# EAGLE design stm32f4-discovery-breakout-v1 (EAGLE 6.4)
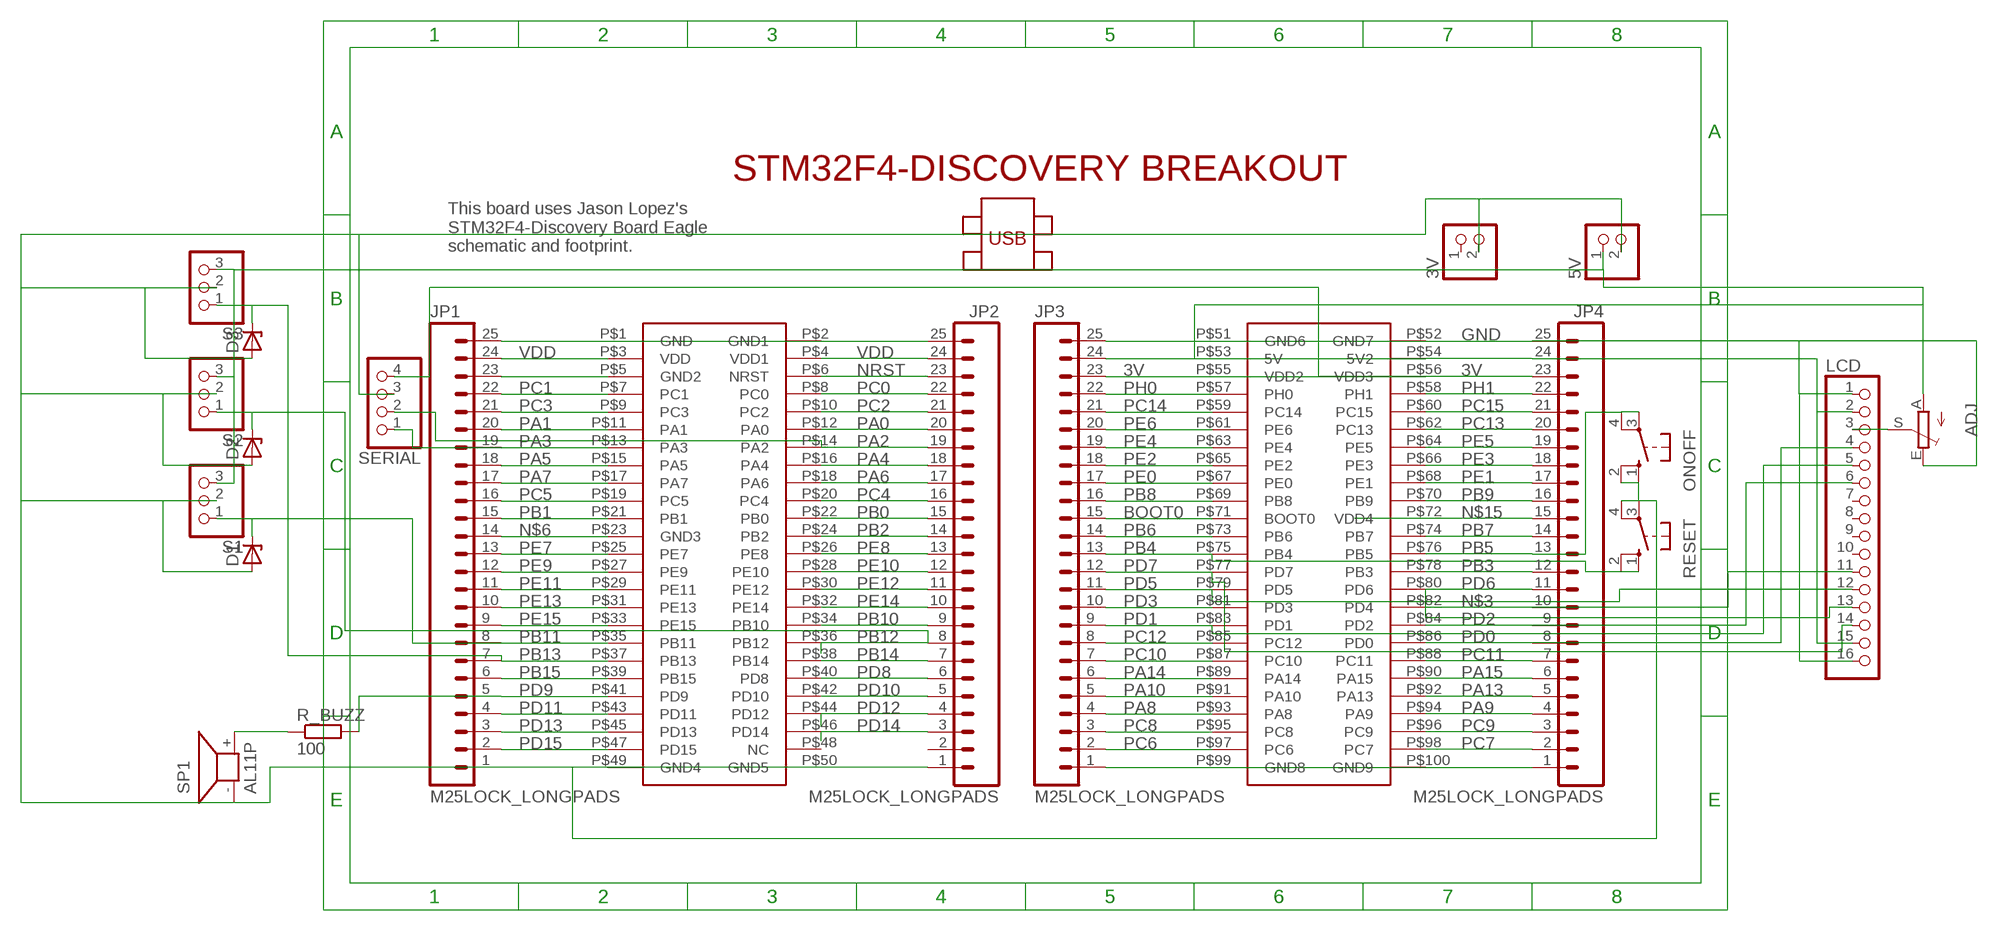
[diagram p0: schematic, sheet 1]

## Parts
3V  PINHD-1X2  [1X02]
5V  PINHD-1X2  [1X02]
ADJ  TRIM_EU-CA6V  [CA6V]
D1  ZENER-DIODEDO35Z10  [DO35Z10]
D2  ZENER-DIODEDO35Z10  [DO35Z10]
D3  ZENER-DIODEDO35Z10  [DO35Z10]
JP1  M25LOCK_LONGPADS  [1X25_LOCK_LONGPADS]
JP2  M25LOCK_LONGPADS  [1X25_LOCK_LONGPADS]
JP3  M25LOCK_LONGPADS  [1X25_LOCK_LONGPADS]
JP4  M25LOCK_LONGPADS  [1X25_LOCK_LONGPADS]
LCD  PINHD-1X16  [1X16]
ONOFF  10-XX  [B3F-10XX]
R_BUZZ  100  R-EU_0204/7  [0204/7]
RESET  10-XX  [B3F-10XX]
S1  PINHD-1X3  [1X03]
S2  PINHD-1X3  [1X03]
S3  PINHD-1X3  [1X03]
SERIAL  PINHD-1X4  [1X04]
SP1  AL11P  [AL11P]
U$1  STM32F4-DISCOVERY  [STM32F4-DISCOVERY]

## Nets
3V: JP3.23 JP4.23 SERIAL.4 U$1.P$55(VDD2) U$1.P$56(VDD3)
+5V: 3V.2 5V.2 D1.A D2.A D3.A JP1.1 JP2.1 ONOFF.1(S) ONOFF.2(S1) RESET.3(P) RESET.4(P1) S1.2 S2.2 S3.2 SERIAL.3 SP1.- U$1.P$49(GND4) U$1.P$50(GND5)
BOOT0: JP3.15 U$1.P$71(BOOT0)
GND: ADJ.E JP3.25 JP4.25 LCD.1 LCD.16 U$1.P$51(GND6) U$1.P$52(GND7)
N$1: R_BUZZ.1 SP1.+
N$2: ADJ.S LCD.3
N$3: JP4.10 LCD.11 U$1.P$82(PD4)
N$4: JP1.25 JP2.25 U$1.P$1(GND) U$1.P$2(GND1)
N$5: JP3.1 JP4.1 U$1.P$99(GND8) U$1.P$100(GND9)
N$6: JP1.14 U$1.P$23(GND3)
N$12: JP1.23 U$1.P$5(GND2)
N$13: 5V.1 ADJ.A JP3.24 JP4.24 LCD.2 LCD.15 S1.3 S2.3 S3.3 U$1.P$53(5V) U$1.P$54(5V2)
N$15: JP4.15 U$1.P$72(VDD4)
NRST: JP2.23 U$1.P$6(NRST)
PA0: JP2.20 U$1.P$12(PA0)
PA1: JP1.20 U$1.P$11(PA1)
PA2: JP2.19 SERIAL.2 U$1.P$14(PA2)
PA3: JP1.19 SERIAL.1 U$1.P$13(PA3)
PA4: JP2.18 U$1.P$16(PA4)
PA5: JP1.18 U$1.P$15(PA5)
PA6: JP2.17 U$1.P$18(PA6)
PA7: JP1.17 U$1.P$17(PA7)
PA8: JP3.4 U$1.P$93(PA8)
PA9: JP4.4 U$1.P$94(PA9)
PA10: JP3.5 U$1.P$91(PA10)
PA13: JP4.5 U$1.P$92(PA13)
PA14: JP3.6 U$1.P$89(PA14)
PA15: JP4.6 U$1.P$90(PA15)
PB0: JP2.15 U$1.P$22(PB0)
PB1: JP1.15 U$1.P$21(PB1)
PB2: JP2.14 U$1.P$24(PB2)
PB3: JP4.12 U$1.P$78(PB3)
PB4: JP3.13 RESET.1(S) RESET.2(S1) U$1.P$75(PB4)
PB5: JP4.13 ONOFF.3(P) ONOFF.4(P1) U$1.P$76(PB5)
PB6: JP3.14 U$1.P$73(PB6)
PB7: JP4.14 U$1.P$74(PB7)
PB8: JP3.16 U$1.P$69(PB8)
PB9: JP4.16 U$1.P$70(PB9)
PB10: JP2.9 U$1.P$34(PB10)
PB11: D1.C JP1.8 S1.1 U$1.P$35(PB11)
PB12: D2.C JP2.8 S2.1 U$1.P$36(PB12)
PB13: D3.C JP1.7 S3.1 U$1.P$37(PB13)
PB14: JP2.7 U$1.P$38(PB14)
PB15: JP1.6 U$1.P$39(PB15)
PC0: JP2.22 U$1.P$8(PC0)
PC1: JP1.22 U$1.P$7(PC1)
PC2: JP2.21 U$1.P$10(PC2)
PC3: JP1.21 U$1.P$9(PC3)
PC4: JP2.16 U$1.P$20(PC4)
PC5: JP1.16 U$1.P$19(PC5)
PC6: JP3.2 U$1.P$97(PC6)
PC7: JP4.2 U$1.P$98(PC7)
PC8: JP3.3 U$1.P$95(PC8)
PC9: JP4.3 U$1.P$96(PC9)
PC10: JP3.7 U$1.P$87(PC10)
PC11: JP4.7 U$1.P$88(PC11)
PC12: JP3.8 U$1.P$85(PC12)
PC13: JP4.20 U$1.P$62(PC13)
PC14: JP3.21 U$1.P$59(PC14)
PC15: JP4.21 U$1.P$60(PC15)
PD0: JP4.8 LCD.4 U$1.P$86(PD0)
PD1: JP3.9 LCD.5 U$1.P$83(PD1)
PD2: JP4.9 LCD.6 U$1.P$84(PD2)
PD3: JP3.10 U$1.P$81(PD3)
PD5: JP3.11 LCD.12 U$1.P$79(PD5)
PD6: JP4.11 LCD.13 U$1.P$80(PD6)
PD7: JP3.12 LCD.14 U$1.P$77(PD7)
PD8: JP2.6 U$1.P$40(PD8)
PD9: JP1.5 R_BUZZ.2 U$1.P$41(PD9)
PD10: JP2.5 U$1.P$42(PD10)
PD11: JP1.4 U$1.P$43(PD11)
PD12: JP2.4 U$1.P$44(PD12)
PD13: JP1.3 U$1.P$45(PD13)
PD14: JP2.3 U$1.P$46(PD14)
PD15: JP1.2 U$1.P$47(PD15)
PE0: JP3.17 U$1.P$67(PE0)
PE1: JP4.17 U$1.P$68(PE1)
PE2: JP3.18 U$1.P$65(PE2)
PE3: JP4.18 U$1.P$66(PE3)
PE4: JP3.19 U$1.P$63(PE4)
PE5: JP4.19 U$1.P$64(PE5)
PE6: JP3.20 U$1.P$61(PE6)
PE7: JP1.13 U$1.P$25(PE7)
PE8: JP2.13 U$1.P$26(PE8)
PE9: JP1.12 U$1.P$27(PE9)
PE10: JP2.12 U$1.P$28(PE10)
PE11: JP1.11 U$1.P$29(PE11)
PE12: JP2.11 U$1.P$30(PE12)
PE13: JP1.10 U$1.P$31(PE13)
PE14: JP2.10 U$1.P$32(PE14)
PE15: JP1.9 U$1.P$33(PE15)
PH0: JP3.22 U$1.P$57(PH0)
PH1: JP4.22 U$1.P$58(PH1)
VDD: JP1.24 JP2.24 U$1.P$3(VDD) U$1.P$4(VDD1)
Unconnected: 3V.1 JP2.2 LCD.7 LCD.8 LCD.9 LCD.10 U$1.P$48(NC)

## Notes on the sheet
- This board uses Jason Lopez's
  STM32F4-Discovery Board Eagle 
  schematic and footprint.

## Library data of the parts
3V 5V = pinhead:PINHD-1X2: PIN HEADER
ADJ = pot:TRIM_EU-: POTENTIOMETER
D1-D3 = diode:ZENER-DIODE: Z-Diode
JP1-JP4 = SparkFun-Connectors:M25: 1x25 .1" header
LCD = pinhead:PINHD-1X16: PIN HEADER
ONOFF RESET = switch-omron:10-XX: OMRON SWITCH; MPN: B3F-1000; OC_FARNELL: 176432; OC_NEWARK: 36M3542
R_BUZZ = rcl:R-EU_: RESISTOR, European symbol
S1-S3 = pinhead:PINHD-1X3: PIN HEADER
SERIAL = pinhead:PINHD-1X4: PIN HEADER
SP1 = buzzer:AL11P: SPEAKER; OC_FARNELL: unknown; OC_NEWARK: unknown
U$1 = STM32F4-DISCOVERY:STM32F4-DISCOVERY

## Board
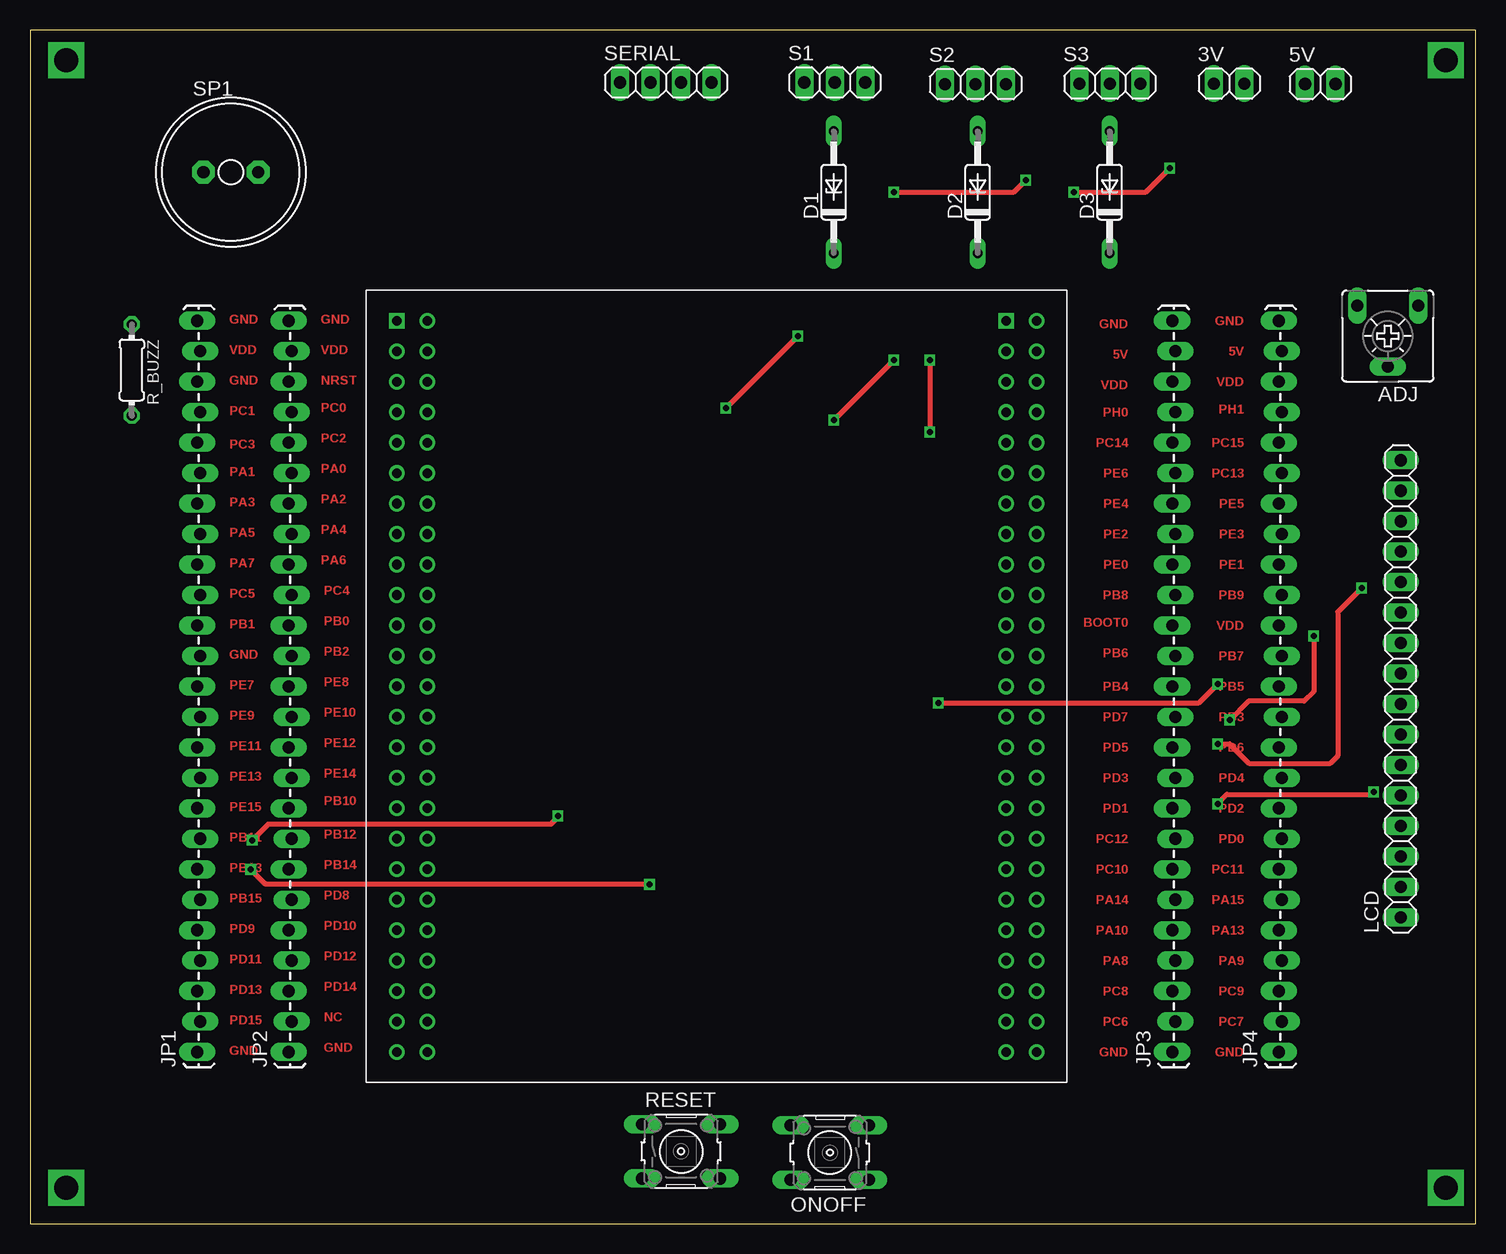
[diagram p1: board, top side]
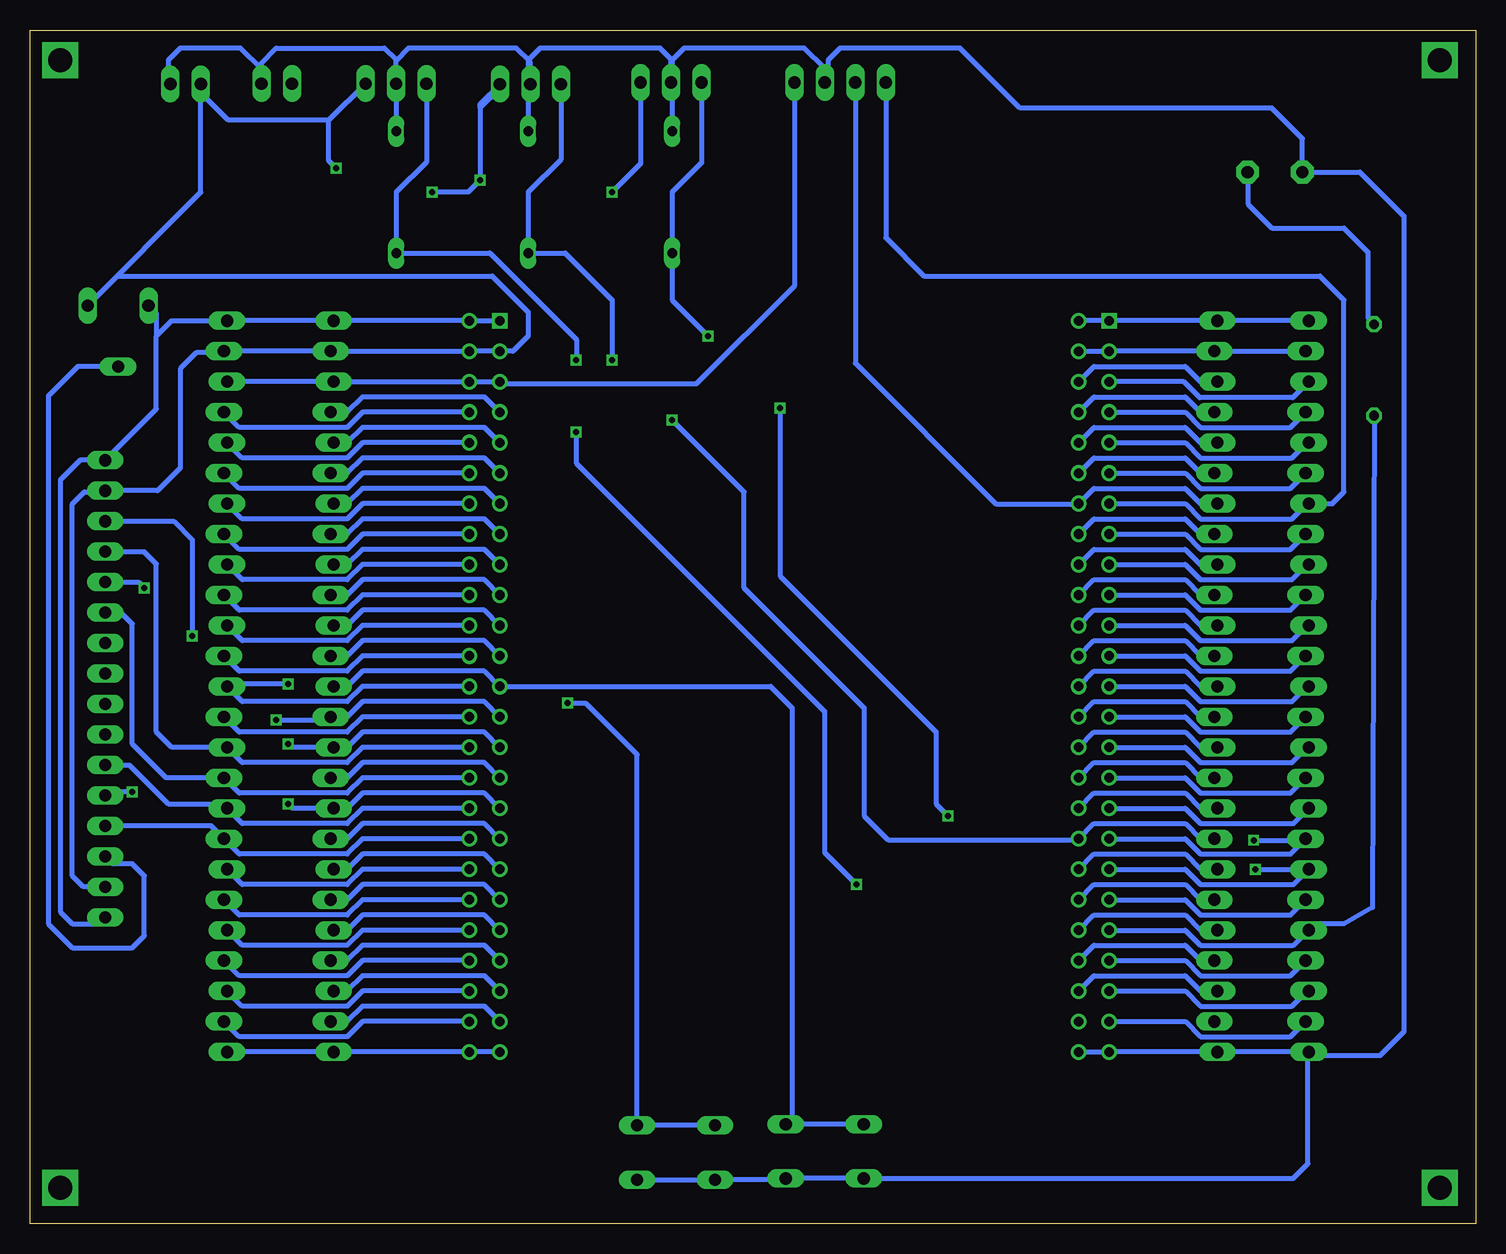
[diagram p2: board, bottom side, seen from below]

Size 120.53 x 99.52 mm. Coordinates in mm from the lower left corner, seen from the top.
Outline: 0,0 120.53,0 120.53,99.52 0,99.52 0,0
Copper layers (1*16): Top 0.035mm / dielectric 1.5mm / Bottom 0.035mm
Design rules "default": minimum track width 10mil, minimum drill 24mil, track to track 8mil, track to pad 8mil, pad to pad 8mil, via to via 8mil, smd to smd 8mil, copper to edge 40mil, drill to drill 8mil, minimum pad ring 10mil, minimum via ring 8mil, stop-mask expansion 4mil, vias tented up to drill 0mil, thermal gap 10mil

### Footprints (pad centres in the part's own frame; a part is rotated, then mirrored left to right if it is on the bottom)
1X02 = drill 1.016 long: 1 -1.27,0; 2 1.27,0
CA6V = drill 1.016 long: A -2.54,-2.54; E 2.54,-2.54; S 0,2.54
DO35Z10 = drill 0.813 long: A 5.08,0; C -5.08,0
1X25_LOCK_LONGPADS = drill 1.016 long: 1 0,0.127; 2 2.54,-0.127; 3 5.08,0.127; 4 7.62,-0.127; 5 10.16,0.127; 6 12.7,-0.127; 7 15.24,0.127; 8 17.78,-0.127; 9 20.32,0.127; 10 22.86,-0.127; 11 25.4,0.127; 12 27.94,-0.127; 13 30.48,0.127; 14 33.02,-0.127; 15 35.56,0.127; 16 38.1,-0.127; 17 40.64,0.127; 18 43.18,-0.127; 19 45.72,0.127; 20 48.26,-0.127; 21 50.8,0.127; 22 53.34,-0.127; 23 55.88,0.127; 24 58.42,-0.127; 25 60.96,0.127
1X16 = drill 1.016 long: 1 -19.05,0; 2 -16.51,0; 3 -13.97,0; 4 -11.43,0; 5 -8.89,0; 6 -6.35,0; 7 -3.81,0; 8 -1.27,0; 9 1.27,0; 10 3.81,0; 11 6.35,0; 12 8.89,0; 13 11.43,0; 14 13.97,0; 15 16.51,0; 16 19.05,0
B3F-10XX = drill 1.016 long: 1 -3.251,2.261; 2 3.251,2.261; 3 -3.251,-2.261; 4 3.251,-2.261
0204/7 = drill 0.813 octagon: 1 -3.81,0; 2 3.81,0
1X03 = drill 1.016 long: 1 -2.54,0; 2 0,0; 3 2.54,0
1X04 = drill 1.016 long: 1 -3.81,0; 2 -1.27,0; 3 1.27,0; 4 3.81,0
AL11P = drill 1.016 pad 1.905 octagon: + 2.286,0; - -2.286,0
STM32F4-DISCOVERY = drill 0.8 square: P$1 -27.94,30.48; P$51 22.86,30.48 | drill 0.8: P$2 -25.4,30.48; P$3 -27.94,27.94; P$4 -25.4,27.94; P$5 -27.94,25.4; P$6 -25.4,25.4; P$7 -27.94,22.86; P$8 -25.4,22.86; P$9 -27.94,20.32; P$10 -25.4,20.32; P$11 -27.94,17.78; P$12 -25.4,17.78; P$13 -27.94,15.24; P$14 -25.4,15.24; P$15 -27.94,12.7; P$16 -25.4,12.7; P$17 -27.94,10.16; P$18 -25.4,10.16; P$19 -27.94,7.62; P$20 -25.4,7.62; P$21 -27.94,5.08; P$22 -25.4,5.08; P$23 -27.94,2.54; P$24 -25.4,2.54; P$25 -27.94,0; P$26 -25.4,0; P$27 -27.94,-2.54; P$28 -25.4,-2.54; P$29 -27.94,-5.08; P$30 -25.4,-5.08; P$31 -27.94,-7.62; P$32 -25.4,-7.62; P$33 -27.94,-10.16; P$34 -25.4,-10.16; P$35 -27.94,-12.7; P$36 -25.4,-12.7; P$37 -27.94,-15.24; P$38 -25.4,-15.24; P$39 -27.94,-17.78; P$40 -25.4,-17.78; P$41 -27.94,-20.32; P$42 -25.4,-20.32; P$43 -27.94,-22.86; P$44 -25.4,-22.86; P$45 -27.94,-25.4; P$46 -25.4,-25.4; P$47 -27.94,-27.94; P$48 -25.4,-27.94; P$49 -27.94,-30.48; P$50 -25.4,-30.48; P$52 25.4,30.48; P$53 22.86,27.94; P$54 25.4,27.94; P$55 22.86,25.4; P$56 25.4,25.4; P$57 22.86,22.86; P$58 25.4,22.86; P$59 22.86,20.32; P$60 25.4,20.32; P$61 22.86,17.78; P$62 25.4,17.78; P$63 22.86,15.24; P$64 25.4,15.24; P$65 22.86,12.7; P$66 25.4,12.7; P$67 22.86,10.16; P$68 25.4,10.16; P$69 22.86,7.62; P$70 25.4,7.62; P$71 22.86,5.08; P$72 25.4,5.08; P$73 22.86,2.54; P$74 25.4,2.54; P$75 22.86,0; P$76 25.4,0; P$77 22.86,-2.54; P$78 25.4,-2.54; P$79 22.86,-5.08; P$80 25.4,-5.08; P$81 22.86,-7.62; P$82 25.4,-7.62; P$83 22.86,-10.16; P$84 25.4,-10.16; P$85 22.86,-12.7; P$86 25.4,-12.7; P$87 22.86,-15.24; P$88 25.4,-15.24; P$89 22.86,-17.78; P$90 25.4,-17.78; P$91 22.86,-20.32; P$92 25.4,-20.32; P$93 22.86,-22.86; P$94 25.4,-22.86; P$95 22.86,-25.4; P$96 25.4,-25.4; P$97 22.86,-27.94; P$98 25.4,-27.94; P$99 22.86,-30.48; P$100 25.4,-30.48

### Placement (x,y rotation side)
3V  99.96,95.05 0 top
5V  107.56,95.02 0 top
ADJ  113.19,74 180 top
D1  67,86 90 top
D2  79,86 90 top
D3  90,86 90 top
JP1  14.06,14.32 90 top
JP2  21.68,14.32 90 top
JP3  95.34,14.32 90 top
JP4  104.23,14.32 90 top
LCD  114.27,44.6 90 top
ONOFF  66.67,5.93 180 top
R_BUZZ  8.48,71.18 270 top
RESET  54.28,6.04 0 top
S1  67.09,95.15 0 top
S2  78.82,95.01 0 top
S3  90.02,95.05 0 top
SERIAL  53,95.15 0 top
SP1  16.75,87.67 0 top
U$1  58.51,44.8 0 top

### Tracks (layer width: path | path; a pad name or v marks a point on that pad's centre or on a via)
3V
  Bottom 0.406: JP4.23 JP3.23 U$1.P$56 U$1.P$55 81.18,70 65,70 56.81,78.19 SERIAL.4
+5V
  Bottom 0.406: U$1.P$50 U$1.P$49 JP2.1 JP1.1 | JP1.1 13.62,14 8,14 6,16 6,84 9.67,87.67 SP1.- 14.46,90.46 17,93 38,93 43,98 53,98 54,97 54,95.42 SERIAL.3 54.27,96.27 56,98 66,98 67,97 67,95.24 S1.2 | S1.2 67.09,97.09 68,98 78,98 79,97 79,95.19 S2.2 | S2.2 78.82,96.82 80,98 89,98 90.02,96.98 S3.2 | ONOFF.1 ONOFF.2 57.63,3.67 RESET.4 RESET.3 15.22,3.77 14,5 14,14.25 JP1.1 | 67.09,91.17 D1.A 67,95.06 S1.2 | S3.2 90.02,97.02 91,98 100,98 101.23,96.77 3V.2 101.23,96.23 103,98 108,98 109,97 109,95.19 5V.2 | S3.2 90,95.03 D3.A | S2.2 79,94.83 D2.A
BOOT0
  Bottom 0.406: U$1.P$71 82.64,51.15 92.8,51.15 94.07,49.88 JP3.15
GND
  Bottom 0.406: U$1.P$51 U$1.P$52 JP3.25 JP4.25 108.72,75.28 110,74 | LCD.1 114.82,25 117,25 118,26 118,62 116.35,63.65 LCD.16 110,67.92 110,74 | ADJ.E 110,75.89 110,74
N$1
  Bottom 0.406: SP1.+ 19,87.64 19,85 17,83 11,83 9,81 9,75.5 R_BUZZ.1
N$2
  Bottom 0.406: ADJ.S 116.54,71.46 119,69 119,25 117,23 112,23 111,24 111,29 112,30 113.64,30 LCD.3
N$3
  Bottom 0.406: U$1.P$82 92.8,37.18 94.07,35.91 103.09,35.91 JP4.10 109.18,37.18 112,40 112,50 113,51 114.22,51 LCD.11
N$4
  Bottom 0.406: JP1.25 JP2.25 U$1.P$1 U$1.P$2
N$5
  Bottom 0.406: U$1.P$99 U$1.P$100 JP3.1 JP4.1
N$6
  Bottom 0.406: U$1.P$23 24.22,47.34 22.95,46.07 15.46,46.07 JP1.14
N$7  (via drill 2)
  other vias: 3,97
N$8  (via drill 2)
  other vias: 118,97
N$9  (via drill 2)
  other vias: 118,3
N$10  (via drill 2)
  other vias: 3,3
N$12
  Bottom 0.406: JP1.23 15.28,68.86 23.02,68.86 24.36,70.2 U$1.P$5
N$13  (via drill 0.5)
  Top 0.406: v87,86 93,86 v95,88 | v72,86 82,86 v83,87
  Bottom 0.406: LCD.2 116.09,28.09 117,29 117,60 116,61 114.38,61 LCD.15 109.89,61.11 108,63 108,71.29 106.68,72.61 104.49,72.61 JP4.24 JP3.24 U$1.P$54 U$1.P$53 80.26,72.74 79,74 79,76 82,79 113.27,79 ADJ.A 106.29,85.98 5V.1 106.29,94.29 104,92 95.62,92 | S3.3 95.62,92 | v95,88 95.62,88.62 95.62,92 | S1.3 69.63,88.37 v72,86 | 83,93 83,93.37 S2.3 81.36,94.64 83,93 | 83,93 v83,87 84,86 v87,86
N$15
  Bottom 0.406: U$1.P$72 92.8,49.88 94.07,48.61 102.84,48.61 JP4.15
NRST
  Bottom 0.406: U$1.P$6 31.84,71.47 24.22,71.47 22.95,70.2 JP2.23
PA0
  Bottom 0.406: U$1.P$12 31.84,63.85 24.22,63.85 22.95,62.58 JP2.20 21.68,62.58
PA1
  Bottom 0.406: U$1.P$11 24.22,62.58 22.95,61.31 15.46,61.31 JP1.20
PA2
  Bottom 0.406: JP2.19 22.95,60.04 24.22,61.31 31.84,61.31 U$1.P$14 33.15,60 40,60 51.73,71.73 SERIAL.2
PA3
  Bottom 0.406: U$1.P$13 24.22,60.04 22.95,58.77 15.33,58.77 14.06,60.04 JP1.19 11.96,60.04 11,61 11,77 13,79 46,79 49.19,82.19 SERIAL.1
PA4
  Bottom 0.406: U$1.P$16 31.84,58.77 24.22,58.77 22.95,57.5 JP2.18 21.68,57.5
PA5
  Bottom 0.406: U$1.P$15 24.22,57.5 22.95,56.23 15.46,56.23 JP1.18
PA6
  Bottom 0.406: U$1.P$18 31.84,56.23 24.22,56.23 22.95,54.96 JP2.17
PA7
  Bottom 0.406: U$1.P$17 24.22,54.96 22.95,53.69 15.33,53.69 14.06,54.96 JP1.17
PA8
  Bottom 0.406: U$1.P$93 82.64,23.21 92.8,23.21 94.07,21.94 JP3.4
PA9
  Bottom 0.406: U$1.P$94 92.8,21.94 94.07,20.67 103.09,20.67 JP4.4
PA10
  Bottom 0.406: U$1.P$91 82.64,25.75 92.8,25.75 94.07,24.48 JP3.5
PA13
  Bottom 0.406: U$1.P$92 92.8,24.48 94.07,23.21 102.84,23.21 JP4.5
PA14
  Bottom 0.406: U$1.P$89 82.64,28.29 92.8,28.29 94.07,27.02 JP3.6
PA15
  Bottom 0.406: U$1.P$90 92.8,27.02 94.07,25.75 103.09,25.75 JP4.6
PB0
  Bottom 0.406: U$1.P$22 31.84,51.15 24.22,51.15 22.95,49.88 JP2.15
PB1
  Bottom 0.406: U$1.P$21 24.22,49.88 22.95,48.61 15.33,48.61 14.06,49.88 JP1.15
PB2
  Bottom 0.406: U$1.P$24 31.84,48.61 24.22,48.61 22.95,47.34 JP2.14
PB3
  Bottom 0.406: U$1.P$78 92.8,42.26 94.07,40.99 103.09,40.99 JP4.12
PB4
  Bottom 0.406: JP3.13 94.07,44.8 92.8,46.07 82.64,46.07 U$1.P$75 58.8,44.8 57,43 57,8.83 RESET.2 RESET.1
PB5  (via drill 0.5)
  Top 0.406: v75.71,43.43 97.43,43.43 v99,45
  Bottom 0.406: U$1.P$76 92.8,44.8 94.07,43.53 102.84,43.53 JP4.13 103.91,45 v99,45 | ONOFF.4 ONOFF.3 69.93,39.11 74.17,43.36 75.64,43.36 v75.71,43.43
PB6
  Bottom 0.406: U$1.P$73 82.64,48.61 92.8,48.61 94.07,47.34 JP3.14
PB7
  Bottom 0.406: U$1.P$74 92.8,47.34 94.07,46.07 103.09,46.07 JP4.14
PB8
  Bottom 0.406: U$1.P$69 82.64,53.69 92.8,53.69 94.07,52.42 JP3.16
PB9
  Bottom 0.406: U$1.P$70 92.8,52.42 94.07,51.15 103.09,51.15 JP4.16
PB10
  Bottom 0.406: U$1.P$34 31.84,35.91 24.22,35.91 22.95,34.64 JP2.9
PB11  (via drill 0.5)
  Top 0.406: v64,74 v58,68 | v44,34 44,33.9 43.4,33.3 19.85,33.3 v18.53,31.98
  Bottom 0.406: U$1.P$35 24.22,32.1 22.95,30.83 15.46,30.83 JP1.8 14.31,31.98 v18.53,31.98 | S1.1 64.55,88.45 67,86 D1.C 67,77 v64,74 | v58,68 58,54 45,41 45,35 v44,34
PB12  (via drill 0.5)
  Top 0.406: v72,72 v67,67
  Bottom 0.406: JP2.8 22.95,32.1 24.22,33.37 31.84,33.37 U$1.P$36 33.21,32 49,32 51,34 51,43 61,53 61,61 v67,67 | S2.1 76.28,88.72 79,86 D2.C 75.92,80.92 72,77 v72,72
PB13  (via drill 0.5)
  Top 0.406: v75,72 v75,66 | v51.65,28.3 19.63,28.3 v18.38,29.55
  Bottom 0.406: U$1.P$37 24.22,29.56 22.95,28.29 15.21,28.29 JP1.7 13.95,29.55 v18.38,29.55 | S3.1 87.48,88.52 90,86 D3.C 82.18,80.92 74.98,73.72 74.98,72.02 v75,72 | v75,66 75,63.43 54.3,42.72 54.3,30.95 v51.65,28.3
PB14
  Bottom 0.406: U$1.P$38 31.84,30.83 24.22,30.83 22.95,29.56 JP2.7
PB15
  Bottom 0.406: U$1.P$39 24.22,27.02 22.95,25.75 15.46,25.75 JP1.6
PC0
  Bottom 0.406: U$1.P$8 31.84,68.93 24.22,68.93 22.95,67.66 JP2.22
PC1
  Bottom 0.406: U$1.P$7 24.22,67.66 22.95,66.39 15.46,66.39 JP1.22
PC2
  Bottom 0.406: U$1.P$10 31.84,66.39 24.22,66.39 22.95,65.12 JP2.21
PC3
  Bottom 0.406: U$1.P$9 24.22,65.12 22.95,63.85 15.33,63.85 14.06,65.12 JP1.21
PC4
  Bottom 0.406: U$1.P$20 31.84,53.69 24.22,53.69 22.95,52.42 JP2.16
PC5
  Bottom 0.406: U$1.P$19 24.22,52.42 22.95,51.15 15.46,51.15 JP1.16
PC6
  Bottom 0.406: U$1.P$97 82.64,18.13 92.8,18.13 94.07,16.86 JP3.2
PC7
  Bottom 0.406: U$1.P$98 92.8,16.86 94.07,15.59 103.09,15.59 JP4.2
PC8
  Bottom 0.406: U$1.P$95 82.64,20.67 92.8,20.67 94.07,19.4 JP3.3
PC9
  Bottom 0.406: U$1.P$96 92.8,19.4 94.07,18.13 102.84,18.13 JP4.3
PC10
  Bottom 0.406: U$1.P$87 82.64,30.83 92.8,30.83 94.07,29.56 JP3.7 95.34,29.56
PC11
  Bottom 0.406: U$1.P$88 92.8,29.56 94.07,28.29 102.84,28.29 JP4.7
PC12
  Bottom 0.406: U$1.P$85 82.64,33.37 92.8,33.37 94.07,32.1 JP3.8
PC13
  Bottom 0.406: U$1.P$62 92.8,62.58 94.07,61.31 103.09,61.31 JP4.20
PC14
  Bottom 0.406: U$1.P$59 82.64,66.39 92.8,66.39 94.07,65.12 JP3.21
PC15
  Bottom 0.406: U$1.P$60 92.8,65.12 94.07,63.85 102.84,63.85 JP4.21
PD0
  Bottom 0.406: U$1.P$86 92.8,32.1 94.07,30.83 103.09,30.83 JP4.8 105.43,33.17 LCD.4
PD1  (via drill 0.5)
  Top 0.406: v99,35 v99,35.01 99.79,35.8 111.8,35.8 v112,36
  Bottom 0.406: U$1.P$83 82.64,35.91 92.8,35.91 94.07,34.64 JP3.9 98.64,34.64 v99,35 | v112,36 113.98,36 LCD.5
PD2
  Bottom 0.406: U$1.P$84 92.8,34.64 94.07,33.37 102.84,33.37 JP4.9 104.47,35 109,35 112.25,38.25 LCD.6
PD3
  Bottom 0.406: U$1.P$81 82.64,38.45 92.8,38.45 94.07,37.18 JP3.10
PD5  (via drill 0.5)
  Top 0.406: v111,53 109,51 109,38.99 108.4,38.39 101.61,38.39 100,40 v99,40
  Bottom 0.406: U$1.P$79 82.64,40.99 92.8,40.99 94.07,39.72 JP3.11 98.72,39.72 v99,40 | LCD.12 111.49,53.49 v111,53
PD6
  Bottom 0.406: U$1.P$80 92.8,39.72 94.07,38.45 102.84,38.45 JP4.11 108.72,39.72 110,41 110,55 111,56 114.24,56 LCD.13
PD7  (via drill 0.5)
  Top 0.406: v107,49 107,44.34 106.23,43.57 101.57,43.57 v100,42
  Bottom 0.406: U$1.P$77 82.64,43.53 92.8,43.53 94.07,42.26 JP3.12 95.73,42 v100,42 | LCD.14 108.57,58.57 107,57 v107,49
PD8
  Bottom 0.406: U$1.P$40 31.84,28.29 24.22,28.29 22.95,27.02 JP2.6
PD9
  Bottom 0.406: U$1.P$41 24.22,24.48 22.95,23.21 15.21,23.21 JP1.5 13.41,25 11,25 8.63,26.37 R_BUZZ.2
PD10
  Bottom 0.406: U$1.P$42 31.84,25.75 24.22,25.75 22.95,24.48 JP2.5
PD11
  Bottom 0.406: U$1.P$43 24.22,21.94 22.95,20.67 15.46,20.67 JP1.4
PD12
  Bottom 0.406: U$1.P$44 31.84,23.21 24.22,23.21 22.95,21.94 JP2.4
PD13
  Bottom 0.406: U$1.P$45 24.22,19.4 22.95,18.13 15.33,18.13 14.06,19.4 JP1.3
PD14
  Bottom 0.406: U$1.P$46 31.84,20.67 24.22,20.67 22.95,19.4 JP2.3
PD15
  Bottom 0.406: U$1.P$47 24.22,16.86 22.95,15.59 15.46,15.59 JP1.2
PE0
  Bottom 0.406: U$1.P$67 82.64,56.23 92.8,56.23 94.07,54.96 JP3.17
PE1
  Bottom 0.406: U$1.P$68 92.8,54.96 94.07,53.69 102.84,53.69 JP4.17
PE2
  Bottom 0.406: U$1.P$65 82.64,58.77 92.8,58.77 94.07,57.5 JP3.18
PE3
  Bottom 0.406: U$1.P$66 92.8,57.5 94.07,56.23 103.09,56.23 JP4.18
PE4
  Bottom 0.406: U$1.P$63 82.64,61.31 92.8,61.31 94.07,60.04 JP3.19
PE5
  Bottom 0.406: U$1.P$64 92.8,60.04 94.07,58.77 102.84,58.77 JP4.19
PE6
  Bottom 0.406: U$1.P$61 82.64,63.85 92.8,63.85 94.07,62.58 JP3.20
PE7
  Bottom 0.406: U$1.P$25 24.22,44.8 22.95,43.53 15.33,43.53 14.06,44.8 JP1.13
PE8
  Bottom 0.406: U$1.P$26 31.84,46.07 24.22,46.07 22.95,44.8 JP2.13
PE9
  Bottom 0.406: U$1.P$27 24.22,42.26 22.95,40.99 15.46,40.99 JP1.12
PE10
  Bottom 0.406: U$1.P$28 31.84,43.53 24.22,43.53 22.95,42.26 JP2.12
PE11
  Bottom 0.406: U$1.P$29 24.22,39.72 22.95,38.45 15.33,38.45 14.06,39.72 JP1.11
PE12
  Bottom 0.406: U$1.P$30 31.84,40.99 24.22,40.99 22.95,39.72 JP2.11
PE13
  Bottom 0.406: U$1.P$31 24.22,37.18 22.95,35.91 15.46,35.91 JP1.10
PE14
  Bottom 0.406: U$1.P$32 31.84,38.45 24.22,38.45 22.95,37.18 JP2.10
PE15
  Bottom 0.406: U$1.P$33 24.22,34.64 22.95,33.37 15.21,33.37 JP1.9
PH0
  Bottom 0.406: U$1.P$57 82.64,68.93 92.8,68.93 94.07,67.66 JP3.22
PH1
  Bottom 0.406: U$1.P$58 92.8,67.66 94.07,66.39 103.09,66.39 JP4.22
VDD
  Bottom 0.406: U$1.P$4 U$1.P$3 JP2.24 JP1.24

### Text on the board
Top: GND | GND | GND | GND | 5V | VDD | VDD | 5V | GND | NRST | VDD | VDD | PC0 | PH0 | PH1 | PC1 | PC3 | PC2 | PC14 | PC15 | PA0 | PE6 | PC13 | PA1 | PA3 | PA2 | PE4 | PE5 | PA5 | PA4 | PE2 | PE3 | PA7 | PA6 | PE0 | PE1 | PC5 | PC4 | PB8 | PB9 | PB1 | PB0 | BOOT0 | VDD | PB6 | GND | PB2 | PB7 | PE7 | PE8 | PB4 | PB5 | PE9 | PE10 | PD7 | PB3 | PE12 | PD5 | PD6 | PE11 | PE13 | PE14 | PD3 | PD4 | PB10 | PD1 | PD2 | PE15 | PB11 | PB12 | PC12 | PD0 | PB14 | PC10 | PC11 | PB13 | PB15 | PD8 | PA14 | PA15 | PD9 | PD10 | PA10 | PA13 | PD11 | PD12 | PA8 | PA9 | PD13 | PD14 | PC8 | PC9 | PD15 | NC | PC6 | PC7 | GND | GND | GND | GND

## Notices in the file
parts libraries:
SparkFun-Connectors: Licensing: Creative Commons ShareAlike 4.0 International - https://creativecommons.org/licenses/by-sa/4.0
